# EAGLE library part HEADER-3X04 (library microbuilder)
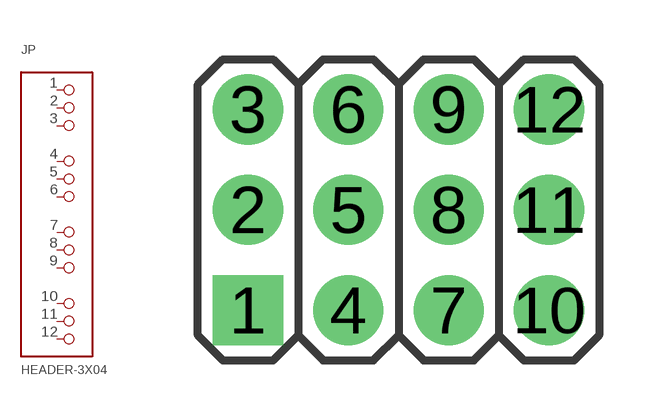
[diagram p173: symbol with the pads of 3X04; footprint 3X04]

Designator prefix JP

## HEADER-3X04  [3X04]
1  1  pas
2  2  pas
3  3  pas
4  4  pas
5  5  pas
6  6  pas
7  7  pas
8  8  pas
9  9  pas
10  10  pas
11  11  pas
12  12  pas

## Footprint 3X04 (pad centres in mm)
drill 1 pad 1.778 square: 1 -3.81,-2.54
drill 1 pad 1.778: 2 -3.81,0; 3 -3.81,2.54; 4 -1.27,-2.54; 5 -1.27,0; 6 -1.27,2.54; 7 1.27,-2.54; 8 1.27,0; 9 1.27,2.54; 10 3.81,-2.54; 11 3.81,0; 12 3.81,2.54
